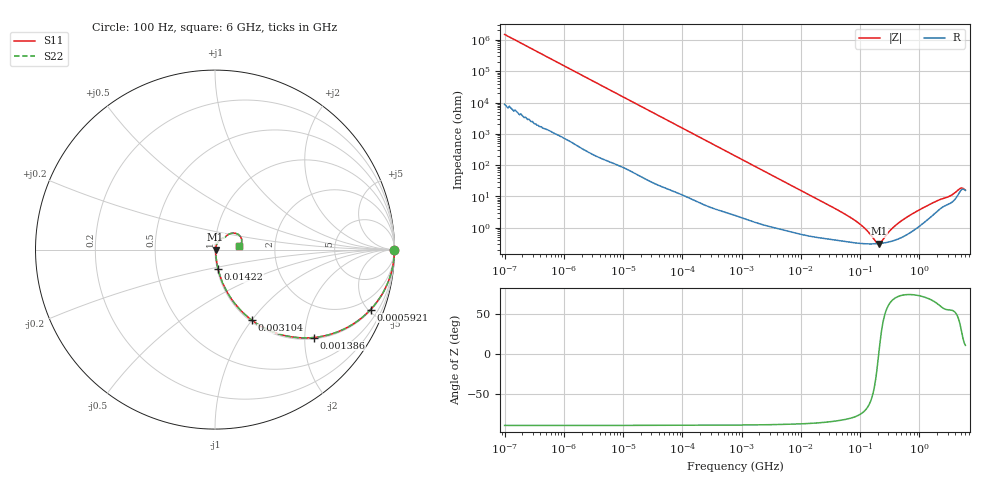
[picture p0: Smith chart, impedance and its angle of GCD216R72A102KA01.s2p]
!Murata Part Number: GCD216R72A102KA01
!These Parameters are Measured in Series Mode Connection
!Data Generated on Jan 08, 2026
!  o--ll--o
!Port1  Port2
!  o------o
!Operation Temp=25[degC], DC Bias Voltage=0[V]
!Freq. Start=100[Hz] Stop=6[GHz] 401[Steps]
# Hz S RI R 50
!Freq.(Hz) S11(Real) S11(Imag) S21(Real) S21(Imag) S12(Real) S12(Imag) S22(Real) S22(Imag)
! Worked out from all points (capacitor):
!   401 points, 100 Hz to 6 GHz, reference 50 ohm
!   read as one part in series: C = 1.07 nF near 109 Hz
!   lowest |Z| = 315 mohm at 208.8 MHz (marker M1)
!   series resonance near 206.8 MHz, so ESL is about 550 pH
!   S11 on the Smith chart (normalised r, x): 100 Hz: open; 592.1 kHz: 1.06, -5.17; 1.386 MHz: 1.03, -2.22; 3.104 MHz: 1.02, -1.00; 14.22 MHz: 1.01, -0.22; 6 GHz: 1.31, +0.06
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100  1 -6.73e-05  4e-07 6.73e-05  4e-07 6.73e-05  1 -6.73e-05
164  1 -0.00011  6e-07 0.00011  6e-07 0.00011  1 -0.00011
2008  1 -0.00134  7.9e-06 0.00134  7.9e-06 0.00134  1 -0.00134
40335  0.9991 -0.0266  0.000869 0.0266  0.000869 0.0266  0.9991 -0.0266
184852  0.9846 -0.1194  0.0154 0.1194  0.0154 0.1194  0.9846 -0.1194
592111  0.8672 -0.3338  0.1328 0.3338  0.1328 0.3338  0.8672 -0.3338
774597  0.7939 -0.3983  0.2061 0.3983  0.2061 0.3983  0.7939 -0.3983
1386327  0.5519 -0.4897  0.4481 0.4897  0.4481 0.4897  0.5519 -0.4897
3103719  0.2048 -0.3929  0.7952 0.3929  0.7952 0.3929  0.2048 -0.3929
5809218  0.0737 -0.2468  0.9263 0.2468  0.9263 0.2468  0.0737 -0.2468
1.422411e7  0.0172 -0.1081  0.9828 0.1081  0.9828 0.1081  0.0172 -0.1081
1.555665e7  0.0152 -0.0991  0.9848 0.0991  0.9848 0.0991  0.0152 -0.0991
8.154455e7  0.00359 -0.0169  0.9964 0.0169  0.9964 0.0169  0.00359 -0.0169
1.220122e8  0.00316 -0.00881  0.9968 0.00881  0.9968 0.00881  0.00316 -0.00881
1.825626e8  0.00308 -0.002  0.9969 0.002  0.9969 0.002  0.00308 -0.002
2.088084e8  0.00313 0.000155  0.9969 -0.000155  0.9969 -0.000155  0.00313 0.000155
3.124326e8  0.0036 0.00679  0.9964 -0.00679  0.9964 -0.00679  0.0036 0.00679
5.112761e8  0.00523 0.0164  0.9948 -0.0164  0.9948 -0.0164  0.00523 0.0164
1.144649e9  0.015 0.0395  0.985 -0.0395  0.985 -0.0395  0.015 0.0395
3.352442e9  0.0635 0.0761  0.9365 -0.0761  0.9365 -0.0761  0.0635 0.0761
4.796499e9  0.1288 0.0848  0.8712 -0.0848  0.8712 -0.0848  0.1288 0.0848
6e9  0.1364 0.0218  0.8636 -0.0218  0.8636 -0.0218  0.1364 0.0218
